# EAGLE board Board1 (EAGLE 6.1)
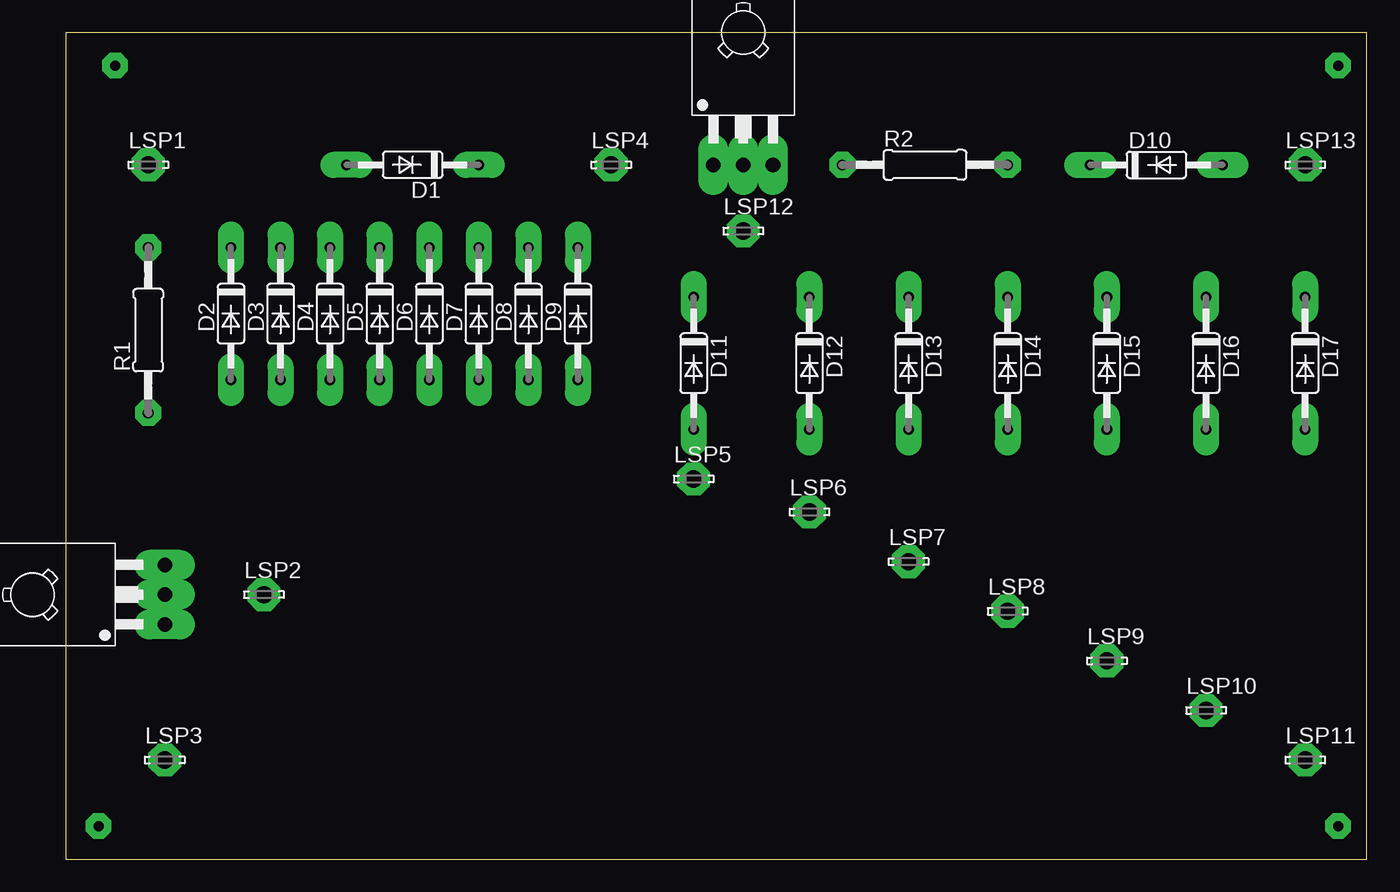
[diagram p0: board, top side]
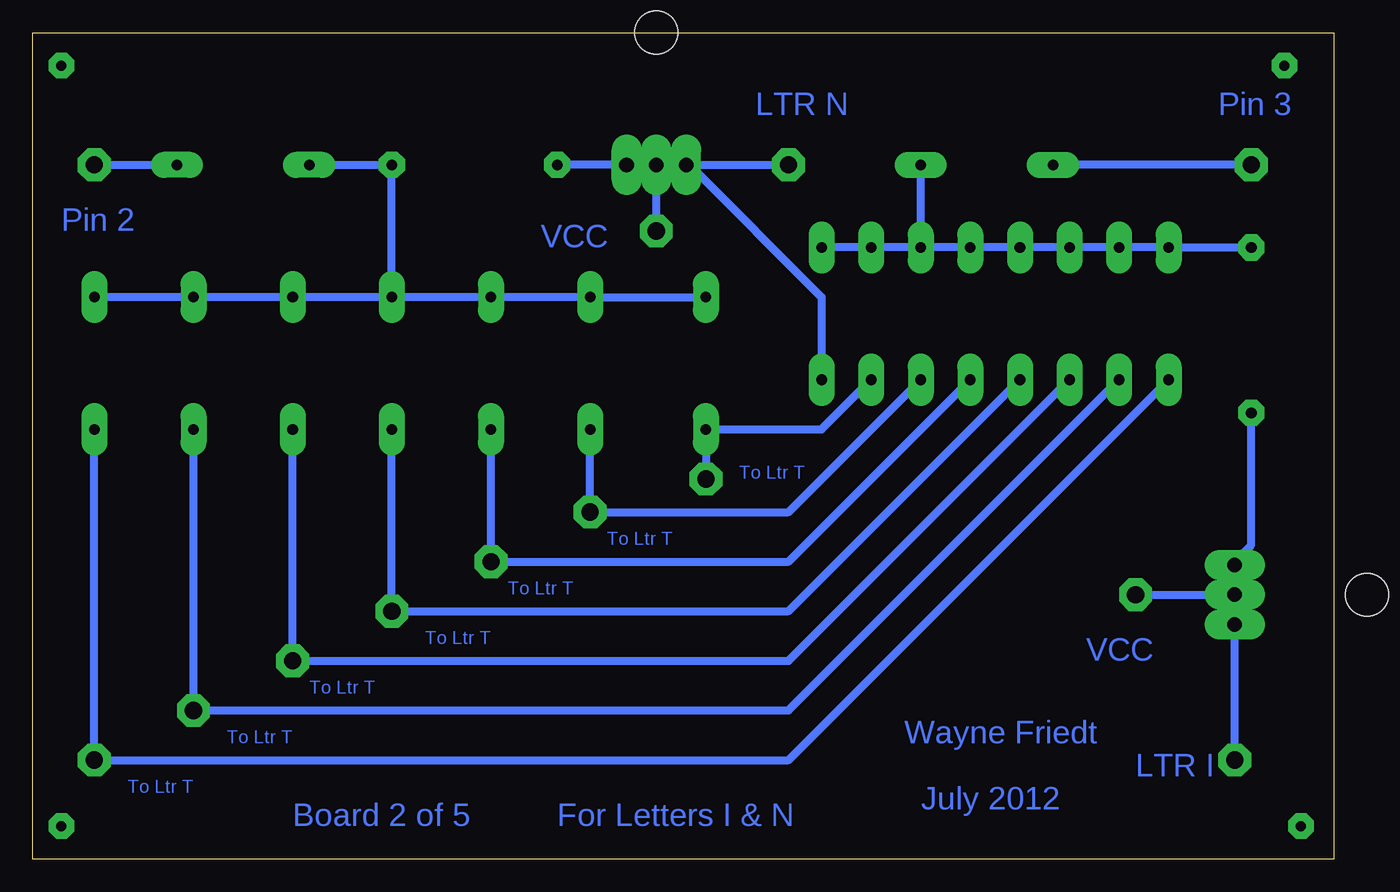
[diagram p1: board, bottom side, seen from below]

Size 100 x 63.49 mm. Coordinates in mm from the lower left corner, seen from the top.
Outline: 0,0 100,0 100,63.49 0,63.49 0,0
Copper layers (1*16): Top 0.035mm / dielectric 1.5mm / Bottom 0.035mm
Design rules: minimum track width 0.6mm, minimum drill 0.8mm, track to track 0.8mm, track to pad 0.8mm, pad to pad 0.45mm, via to via 0.8mm, smd to smd 8mil, copper to edge 10mil, drill to drill 8mil, minimum pad ring 0.6mm, minimum via ring 0.6mm, stop-mask expansion 0mil, vias tented up to drill 0mil, thermal gap 10mil

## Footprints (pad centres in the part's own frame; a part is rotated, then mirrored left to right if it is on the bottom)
DO35-10 = drill 0.813 long: A 5.08,0; C -5.08,0
LSP13 = drill 1.321 pad 2.159 octagon: MP 0,0
0207/12 = drill 0.813 octagon: 1 -6.35,0; 2 6.35,0
TO126 = drill 1.118 long: 1 -2.286,-5.08; 2 0,-5.08; 3 2.286,-5.08 | hole 3.302: 0,5.08

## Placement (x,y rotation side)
D1  1N4148DO35-10  [DO35-10]  26.67,53.34 180 top
D2  1N4148DO35-10  [DO35-10]  12.7,41.91 270 top
D3  1N4148DO35-10  [DO35-10]  16.51,41.91 270 top
D4  1N4148DO35-10  [DO35-10]  20.32,41.91 270 top
D5  1N4148DO35-10  [DO35-10]  24.13,41.91 270 top
D6  1N4148DO35-10  [DO35-10]  27.94,41.91 270 top
D7  1N4148DO35-10  [DO35-10]  31.75,41.91 270 top
D8  1N4148DO35-10  [DO35-10]  35.56,41.91 270 top
D9  1N4148DO35-10  [DO35-10]  39.37,41.91 270 top
D10  1N4148DO35-10  [DO35-10]  83.82,53.34 0 top
D11  1N4148DO35-10  [DO35-10]  48.26,38.1 270 top
D12  1N4148DO35-10  [DO35-10]  57.15,38.1 270 top
D13  1N4148DO35-10  [DO35-10]  64.77,38.1 270 top
D14  1N4148DO35-10  [DO35-10]  72.39,38.1 270 top
D15  1N4148DO35-10  [DO35-10]  80.01,38.1 270 top
D16  1N4148DO35-10  [DO35-10]  87.63,38.1 270 top
D17  1N4148DO35-10  [DO35-10]  95.25,38.1 270 top
LSP1  LSP13  [LSP13]  6.35,53.34 0 top
LSP2  LSP13  [LSP13]  15.24,20.32 0 top
LSP3  LSP13  [LSP13]  7.62,7.62 0 top
LSP4  LSP13  [LSP13]  41.91,53.34 0 top
LSP5  LSP13  [LSP13]  48.26,29.21 0 top
LSP6  LSP13  [LSP13]  57.15,26.67 0 top
LSP7  LSP13  [LSP13]  64.77,22.86 0 top
LSP8  LSP13  [LSP13]  72.39,19.05 0 top
LSP9  LSP13  [LSP13]  80.01,15.24 0 top
LSP10  LSP13  [LSP13]  87.63,11.43 0 top
LSP11  LSP13  [LSP13]  95.25,7.62 0 top
LSP12  LSP13  [LSP13]  52.07,48.26 0 top
LSP13  LSP13  [LSP13]  95.25,53.34 0 top
R1  [0207/12]  6.35,40.64 90 top
R2  [0207/12]  66.04,53.34 0 top
T1  BD139  [TO126]  2.54,20.32 90 top
T2  BD139  [TO126]  52.07,58.42 0 top

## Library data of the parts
D1-D17 = diode
LSP1-LSP13 = solpad
R1 R2 = resistor
T1 T2 = transistor-neu-to92

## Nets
N$1: R1.1 T1.3
N$2: D1.C D2.C D3.C D4.C D5.C D6.C D7.C D8.C D9.C R1.2
N$3: D10.C D11.C D12.C D13.C D14.C D15.C D16.C D17.C R2.2
N$4: LSP2.MP T1.2
N$5: R2.1 T2.3
N$6: D10.A LSP13.MP
N$7: LSP12.MP T2.2
N$10: D2.A D17.A LSP11.MP
N$11: LSP3.MP T1.1
N$13: D1.A LSP1.MP
N$14: D9.A LSP4.MP T2.1
N$15: D8.A D11.A LSP5.MP
N$16: D7.A D12.A LSP6.MP
N$17: D6.A D13.A LSP7.MP
N$18: D5.A D14.A LSP8.MP
N$19: D4.A D15.A LSP9.MP
N$20: D3.A D16.A LSP10.MP

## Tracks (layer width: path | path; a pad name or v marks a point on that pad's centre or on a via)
N$1
  Bottom 0.6: R1.1 6.35,24.13 7.62,22.86 T1.3
N$2
  Bottom 0.6: R1.2 D2.C D3.C D4.C D5.C D6.C D7.C | D7.C D8.C D9.C | D7.C D1.C
N$3
  Bottom 0.6: D11.C D12.C D13.C D14.C | D14.C D15.C D16.C D17.C | D10.C R2.2 D14.C
N$4
  Bottom 0.6: LSP2.MP T1.2
N$5
  Bottom 0.6: T2.3 R2.1
N$6
  Bottom 0.6: LSP13.MP D10.A
N$7
  Bottom 0.6: LSP12.MP T2.2
N$8  (via drill 0.76)
  other vias: 3.81,60.96 97.79,60.96 97.79,2.54 2.54,2.54
N$10
  Bottom 0.6: D2.A 41.91,7.62 LSP11.MP D17.A
N$11
  Bottom 0.6: LSP3.MP T1.1
N$13
  Bottom 0.6: LSP1.MP D1.A
N$14
  Bottom 0.6: D9.A 39.37,43.18 49.53,53.34 | 49.53,53.34 T2.1 | 49.53,53.34 LSP4.MP
N$15
  Bottom 0.6: D8.A 39.37,33.02 D11.A LSP5.MP
N$16
  Bottom 0.6: D7.A 41.91,26.67 LSP6.MP D12.A
N$17
  Bottom 0.6: D6.A 41.91,22.86 LSP7.MP D13.A
N$18
  Bottom 0.6: D5.A 41.91,19.05 LSP8.MP D14.A
N$19
  Bottom 0.6: D4.A 41.91,15.24 LSP9.MP D15.A
N$20
  Bottom 0.6: D3.A 41.91,11.43 LSP10.MP D16.A

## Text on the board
Bottom: Pin 3 | LTR N | Pin 2 | VCC | To Ltr T | To Ltr T | To Ltr T | To Ltr T | VCC | To Ltr T | Wayne Friedt | To Ltr T | LTR I | To Ltr T | July 2012 | For Letters I & N | Board 2 of 5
